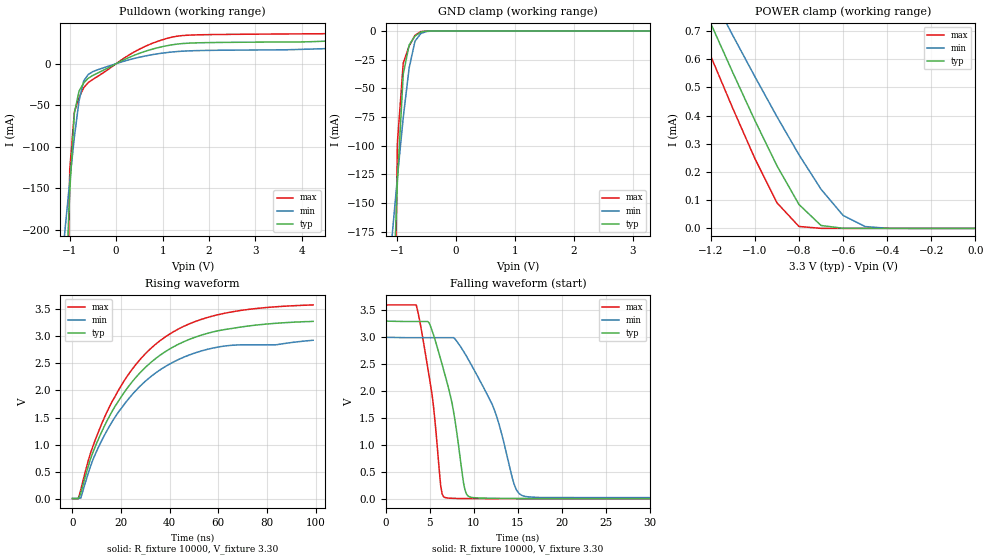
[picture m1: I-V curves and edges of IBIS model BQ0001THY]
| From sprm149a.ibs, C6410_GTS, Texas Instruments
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| Reserved Pins
| B11   RESERVED
| B12   RESERVED
| C10   RESERVED
| D7   RESERVED
| D8   RESERVED
| U4   RESERVED
| F3   RESERVED
| C8   RESERVED
|****** ****   ***** *****   ******  Buffer Models  ***************************
[Model]   BQ0001THY
|  I2C  I/O BUFFER
Model_type   I/O_open_sink
Vinh = 2.00
Vinl = 0.80
Enable   Active-Low
Polarity   Non-Inverting
| signals   A, GZ, Y
Vmeas = 1.5
|   typ   min   max
C_comp   3.010p   2.982p   3.113p
|   typ   min   max
[Temperature Range]   25   -40   125
|   typ   min   max
[Voltage Range]   3.30V   3.00V   3.60V
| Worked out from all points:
|   slope of the pulldown table from 0 to 0.495 V, typ, clamps not added: 40.1 ohm
|   GND clamp passes 1 mA (typ) near -0.60 V on its own axis
|   POWER clamp passes 1 mA (typ) near -1.35 V on its own axis
|   falling waveform, R_fixture 10000, V_fixture 3.30: 20-80 % time 2.38ns typ, 4.04ns min, 1.67ns max; typ from 3.3 V to 0.011 V
|   rising waveform, R_fixture 10000, V_fixture 3.30: 20-80 % time 28.3ns typ, 27.5ns min, 27.9ns max; typ from 0.011 V to 3.27 V
[Pulldown]
|   Voltage   I(typ)   I(min)   I(max)
-3.3V     -4.063A    -1.593A    -14.67A
-1.1V     -294mA     -199mA     -512.7mA
-1V       -153.6mA   -141.5mA   -127.5mA
-900mV    -59.38mA   -88.28mA   -58.05mA
-800mV    -33.14mA   -44.79mA   -41.02mA
-700mV    -23.32mA   -20.88mA   -29.03mA
-600mV    -17.47mA   -12.92mA   -22.67mA
-500mV    -14.14mA   -9.52mA    -18.92mA
500mV     12.44mA    7.712mA    17.41mA
900mV     19.22mA    11.91mA    26.99mA
1.3V      23.44mA    14.5mA     32.94mA
6.6V      31.34mA    21.66mA    40.76mA
[GND_clamp]
|   Voltage   I(typ)   I(min)   I(max)
-3.3V     -4.062A    -1.593A    -14.67A
-1.1V     -272.2mA   -185mA     -484.5mA
-1V       -132.4mA   -128mA     -98mA
-900mV    -37.7mA    -75.42mA   -27.94mA
-800mV    -12.21mA   -32.29mA   -13.11mA
-700mV    -4.383mA   -8.804mA   -3.73mA
-600mV    -840.8uA   -2.113mA   -413.8uA
-500mV    -76.47uA   -376.6uA   -19.23uA
-400mV    -4.269uA   -46.15uA   -428.2nA
3.3V      177.6pA    31.97nA    177.6pA
[POWER_clamp]
|   Voltage   I(typ)   I(min)   I(max)
-3.3V     4.599mA    4.102mA    4.747mA
-1.3V     905.1uA    983.6uA    800.7uA
-1.2V     727.5uA    833.2uA    611.3uA
-1.1V     552.9uA    684.7uA    425.8uA
-1V       383.1uA    538.7uA    248.1uA
-900mV    222.6uA    396.7uA    91.01uA
-800mV    84.79uA    261.3uA    6.786uA
-700mV    10.3uA     138.9uA    73.81nA
-600mV    329.7nA    46.05uA    888.2pA
-500mV    8.438nA    6.46uA     266.4pA
-400mV    399.7pA    466.9nA    222pA
0V        1pA        1pA        1pA
[Ramp]
|   I(typ)   I(min)   I(max)
dV/dt_r   0.001/10.000n   0.001/20.000n   0.001/5.000n
dV/dt_f   1.973/2.375n   1.790/4.037n   2.155/1.664n
[Falling Waveform]
R_fixture = 10000
V_fixture = 3.30
V_fixture_min = 3.00
V_fixture_max = 3.60
|  pd_on
|  TIME   V(typ)   V(min)   V(max)
0s        3.3V       3V         3.6V
3.489ns   3.293V     2.993V     3.596V
5.279ns   3.124V     2.993V     1.939V
6.255ns   2.594V     2.993V     259.4mV
6.905ns   2.208V     2.993V     24.64mV
9.182ns   98.78mV    2.651V     11.07mV
12.44ns   15.08mV    1.62V      9.088mV
14.71ns   12.67mV    228.1mV    8.836mV
15.85ns   12.13mV    51.1mV     8.791mV
99ns      11.14mV    16.4mV     8.68mV
[Rising Waveform]
R_fixture = 10000
V_fixture = 3.30
V_fixture_min = 3.00
V_fixture_max = 3.60
|  pd_off
|  TIME   V(typ)   V(min)   V(max)
0s        11.13mV    16.39mV    8.679mV
2.432ns   11.13mV    16.39mV    8.679mV
3.417ns   108.9mV    20.54mV    173.3mV
8.344ns   852.7mV    715.9mV    964.3mV
16.23ns   1.608V     1.417V     1.789V
25.09ns   2.186V     1.949V     2.419V
34.94ns   2.61V      2.343V     2.874V
45.78ns   2.893V     2.61V      3.176V
59.58ns   3.092V     2.793V     3.387V
99ns      3.268V     2.921V     3.57V
